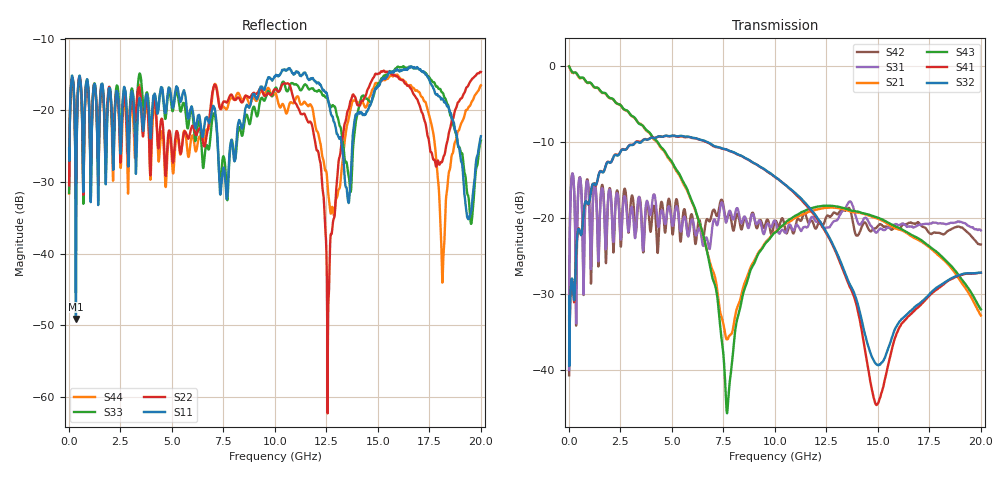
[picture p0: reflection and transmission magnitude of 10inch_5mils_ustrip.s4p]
! FILE: C:\Archive\FR4 ustrip trace\5mils\10inch_5mils_ustrip.s4p
# MHz S DB R 50.00
! FREQ  S11  S12  S13  S14
!  S21  S22  S23  S24
!  S31  S32  S33  S34
!  S41  S42  S43  S44
!  DB  ANG  DB  ANG  DB  ANG  DB  ANG
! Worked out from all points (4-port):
!   2000 points, 10 MHz to 20 GHz, reference 50 ohm
!   strongest paths, dB at 10 MHz, 5.01 GHz, 10.01 GHz, 15.01 GHz, 20 GHz:
!     S32: -30.3, -9.2, -14.6, -39.4, -27.2
!     S41: -33.0, -9.2, -14.7, -44.4, -27.2
!     S43: -0.1, -12.7, -22.0, -20.0, -32.0
!     S21: -0.1, -12.8, -21.9, -20.1, -32.9
!     S31: -40.0, -20.9, -20.4, -21.7, -21.7
!     S42: -40.7, -21.8, -20.4, -21.1, -23.5
!   lowest |S11| = -49.1 dB at 340 MHz (marker M1), VSWR 1.01, Z = 50.4 + j0.0291 ohm
!   |S11| at or under -10 dB: start of sweep to end of sweep
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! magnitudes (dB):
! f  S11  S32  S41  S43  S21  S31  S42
! 10 MHz  -25.3  -30.3  -33.0  -0.1  -0.1  -40.0  -40.7
! 340 MHz  -49.1  -25.5  -25.5  -0.9  -1.0  -31.6  -31.4
! 7.69 GHz  -31.9  -11.1  -11.1  -45.6  -36.0  -20.2  -20.0
! 12.59 GHz  -18.7  -22.3  -22.5  -18.4  -18.7  -21.3  -19.7
! 13.75 GHz  -25.0  -29.3  -29.7  -19.1  -19.2  -18.2  -20.0
! 18.15 GHz  -18.4  -28.7  -28.8  -25.2  -25.4  -20.7  -22.2
! 20 GHz  -23.6  -27.2  -27.2  -32.0  -32.9  -21.7  -23.5
